(* Logix 5000 AddOnInstructionDefinition export Banner_K50Audible_PD_v4; software revision 33.00 *)

TYPE Banner_K50Audible_Advanced_PD_v4 :   // K50 Pro Audible Advanced
STRUCT
   PDI_Output_State : SINT;   // 0 = Inactive,1 = Active
   PDO_Animation : SINT;   // 0 = Off, 1 = Steady, 2 = Flash, 3 = 2 Color Flash, 4 = 50/50, 5 = 50/50 Rotate, 6 = Chase, 7 = Intensity Sweep, 8 = Color Sweep, 9 Sequence, 10 = Wave, 11 = Double Wave
   PDO_Direction : SINT;   // 0 = CCW, 1 = CW
   PDO_Pattern : SINT;   // 0 = Slow, 1 = Strobe, 2 = 3 Pulse, 3 = SOS, 4 = Random
   PDO_Speed : SINT;   // 0 = Slow, 1 = Medium, 2 = Fast, 3 = Custom
   PDO_Audio_Feedback : SINT;   // 0 = Off, 1 = On, 2 = Animation Pattern, 3 = Advanced Audible
   PDO_Off_Delay_Type : SINT;   // 0 = Leading Edge, 1 = Trailing Edge
   PDO_Off_Delay : DINT;   // 0 to 65535. Length of time before device returns to touch inactive after button press.
   PDO_Static_Sequence : SINT;   // 0 to 255. Value describing LED position
   PDO_Sequence_Start_Location : SINT;   // 0 = LED1, 1 = LED2, 2 = LED3, 3 = LED4, 4 = LED5, 5 = LED6, 6 = LED7, 7 = LED8
   PDO_Color_1 : SINT;   // 0 = Green, 1 = Red, 2 = Orange, 3 = Amber, 4 = Yellow, 5 = Lime Green, 6 = Spring Green, 7 = Cyan, 8 = Sky Blue, 9 = Blue, 10 = Violet, 11 = Magenta, 12 = Rose, 13 = White, 14 = Custom 1, 15 = Custom 2
   PDO_Color_1_Intensity : SINT;   // 0 = High, 1 = Medium, 2 = Low, 3 = Off, 4 = Custom
   PDO_Color_2 : SINT;   // 0 = Green, 1 = Red, 2 = Orange, 3 = Amber, 4 = Yellow, 5 = Lime Green, 6 = Spring Green, 7 = Cyan, 8 = Sky Blue, 9 = Blue, 10 = Violet, 11 = Magenta, 12 = Rose, 13 = White, 14 = Custom 1, 15 = Custom 2.
   PDO_Color_2_Intensity : SINT;   // 0 = High, 1 = Medium, 2 = Low, 3 = Off, 4 = Custom
   PDO_Audio_Volume : SINT;   // 1 = Low, 3 = High
   PDO_Audio_Type : SINT;   // 0 = Pulse, 1 = Wobble, 2 = Strobe, 3 = Whoop, 4 = Stacatto, 5 = Siren, 6 = Continuous 1, 7 = Continuous 2, 9 = Jingle, 10 = Melody 1, 11 = Melody 2, 12 = Melody 3, 13 Custom
END_STRUCT
END_TYPE

TYPE Banner_K50Audible_Four_PD_v4 :   // K50 Pro Audible Four State Full Logic
STRUCT
   PDI_Output_State : SINT;   // 0 = Inactive,1 = Active
   PDI_State : SINT;   // 0 = State 1, 1 = State 2, 2 = State 3, 3 = State 4
   PDO_Job_Input : SINT;   // 0 = State 1, 1 = State 2, 2 = State 3, 3 = State 4
END_STRUCT
END_TYPE

TYPE Banner_K50Audible_LED_v4 :   // LED Control Process Data for a K50 Pro Audible.
STRUCT
   Output_State : SINT;   // 0 = Inactive, 1 = Active.
   LED_1_Color : SINT;   // 0 = Green, 1 = Red, 2 = Orange, 3 = Amber, 4 = Yellow, 5 = Lime Green, 6 = Spring Green, 7 = Cyan, 8 = Sky Blue, 9 = Blue, 10 = Violet, 11 = Magenta, 12 = Rose, 13 = White, 14 = Custom 1, 15 = Custom 2.
   LED_1_Intensity : SINT;   // 0 to 10 (0 to 100%).
   LED_2_Color : SINT;   // 0 = Green, 1 = Red, 2 = Orange, 3 = Amber, 4 = Yellow, 5 = Lime Green, 6 = Spring Green, 7 = Cyan, 8 = Sky Blue, 9 = Blue, 10 = Violet, 11 = Magenta, 12 = Rose, 13 = White, 14 = Custom 1, 15 = Custom 2.
   LED_2_Intensity : SINT;   // 0 to 10 (0 to 100%).
   LED_3_Color : SINT;   // 0 = Green, 1 = Red, 2 = Orange, 3 = Amber, 4 = Yellow, 5 = Lime Green, 6 = Spring Green, 7 = Cyan, 8 = Sky Blue, 9 = Blue, 10 = Violet, 11 = Magenta, 12 = Rose, 13 = White, 14 = Custom 1, 15 = Custom 2.
   LED_3_Intensity : SINT;   // 0 to 10 (0 to 100%).
   LED_4_Color : SINT;   // 0 = Green, 1 = Red, 2 = Orange, 3 = Amber, 4 = Yellow, 5 = Lime Green, 6 = Spring Green, 7 = Cyan, 8 = Sky Blue, 9 = Blue, 10 = Violet, 11 = Magenta, 12 = Rose, 13 = White, 14 = Custom 1, 15 = Custom 2.
   LED_4_Intensity : SINT;   // 0 to 10 (0 to 100%).
   LED_5_Color : SINT;   // 0 = Green, 1 = Red, 2 = Orange, 3 = Amber, 4 = Yellow, 5 = Lime Green, 6 = Spring Green, 7 = Cyan, 8 = Sky Blue, 9 = Blue, 10 = Violet, 11 = Magenta, 12 = Rose, 13 = White, 14 = Custom 1, 15 = Custom 2.
   LED_5_Intensity : SINT;   // 0 to 10 (0 to 100%).
   LED_6_Color : SINT;   // 0 = Green, 1 = Red, 2 = Orange, 3 = Amber, 4 = Yellow, 5 = Lime Green, 6 = Spring Green, 7 = Cyan, 8 = Sky Blue, 9 = Blue, 10 = Violet, 11 = Magenta, 12 = Rose, 13 = White, 14 = Custom 1, 15 = Custom 2.
   LED_6_Intensity : SINT;   // 0 to 10 (0 to 100%).
   LED_7_Color : SINT;   // 0 = Green, 1 = Red, 2 = Orange, 3 = Amber, 4 = Yellow, 5 = Lime Green, 6 = Spring Green, 7 = Cyan, 8 = Sky Blue, 9 = Blue, 10 = Violet, 11 = Magenta, 12 = Rose, 13 = White, 14 = Custom 1, 15 = Custom 2.
   LED_7_Intensity : SINT;   // 0 to 10 (0 to 100%).
   LED_8_Color : SINT;   // 0 = Green, 1 = Red, 2 = Orange, 3 = Amber, 4 = Yellow, 5 = Lime Green, 6 = Spring Green, 7 = Cyan, 8 = Sky Blue, 9 = Blue, 10 = Violet, 11 = Magenta, 12 = Rose, 13 = White, 14 = Custom 1, 15 = Custom 2.
   LED_8_Intensity : SINT;   // 0 to 10 (0 to 100%).
   Audio_Feedback : SINT;   // 0 = Off, 1 = On, 2 = Pattern, 3 = Advanced Audible
   Audio_Volume : SINT;   // 1 = Low, 3 = High
   Audio_Type : SINT;   // 0 = Pulse, 1 = Wobble, 2 = Strobe, 3 = Whoop, 4 = Stacatto, 5 = Siren, 6 = Continuous 1, 7 = Continuous 2, 9 = Jingle, 10 = Melody 1, 11 = Melody 2, 12 = Melody 3, 13 Custom
END_STRUCT
END_TYPE

TYPE Banner_K50Audible_Multi_PD_v4 :   // K50 Pro Audible Multicolor Process Data
STRUCT
   PDI_Output_State : SINT;   // 0 = Inactive,1 = Active
   PDI_State : SINT;   // 0 = State 1, 1 = State 2, 2 = State 3, 3 = State 4
   PDO_State : SINT;   // 0 = State 1, 1 = State 2, 2 = State 3, 3 = State 4
END_STRUCT
END_TYPE

TYPE Banner_K50Audible_PDIO_v4 :   // UDT that records the converted prcoess data.
STRUCT
   PD_MultiColor_State : Banner_K50Audible_Multi_PD_v4;   // Only active when Operation Mode set to 0. State tells the light which of the four states it should be in. 0 = State 1, 1 = State 2, 2 = State 3, 3 = State 4.
   PD_FourState_Job_Input : Banner_K50Audible_Four_PD_v4;   // Only active when Operation Mode set to 1. Job Input tells the light how it should behave. 0 - Off, 1 = ON
   PD_Advanced : Banner_K50Audible_Advanced_PD_v4;   // Only active when Operation Mode set to 2.
   PD_LED : Banner_K50Audible_LED_v4;   // Only active when Operation Mode set to 3.
   PDO_DT : SINT[10];
   PDI_DT : SINT[2];
END_STRUCT
END_TYPE

ADD_ON_INSTRUCTION Banner_K50Audible_PD_v4   (* revision 4.0, vendor Banner Engineering *)
// Takes the raw SINT information and converts that data into actual information.
VAR_IN_OUT
   PDIO : Banner_K50Audible_PDIO_v4; {required}
END_VAR
VAR_INPUT
   Operation_Mode : SINT; {required}   // Linked from Parameters AOI or entered manually.
   Byte_Swap : BOOL; {required}
END_VAR
VAR
   PDO_Temp : SINT[10]; {access None}
   PDI_Temp : SINT[2]; {access None}
END_VAR

ROUTINE Logic   (* ladder *)
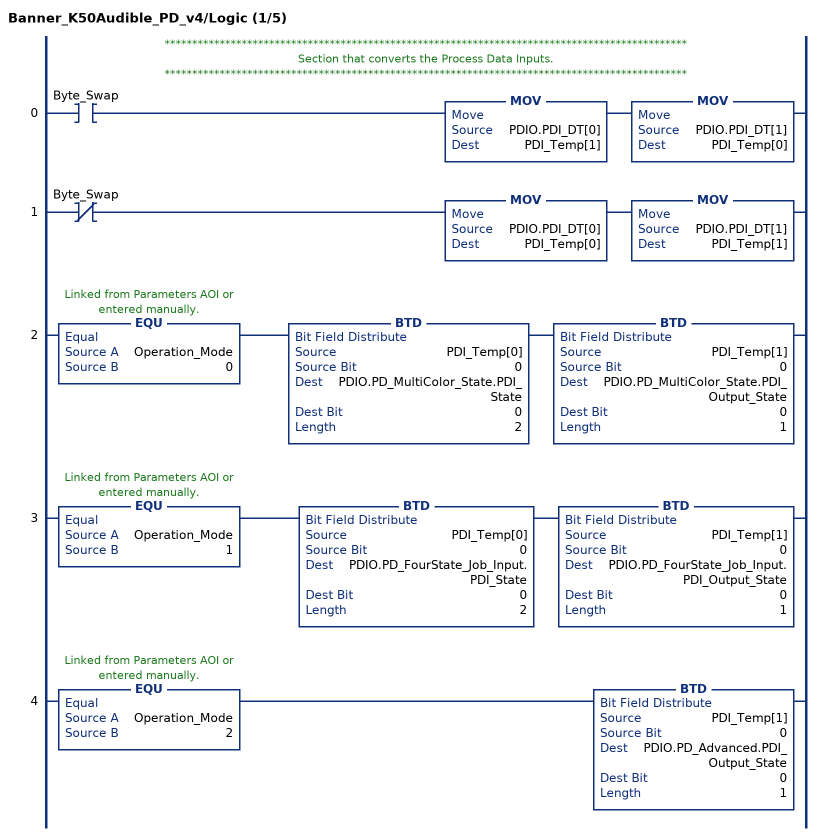
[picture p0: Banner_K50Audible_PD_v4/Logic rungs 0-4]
   // ***********************************************************************************************
   // Section that converts the Process Data Inputs.
   // ***********************************************************************************************
   0: XIC(Byte_Swap)MOV(PDIO.PDI_DT[0],PDI_Temp[1])MOV(PDIO.PDI_DT[1],PDI_Temp[0]);
   1: XIO(Byte_Swap)MOV(PDIO.PDI_DT[0],PDI_Temp[0])MOV(PDIO.PDI_DT[1],PDI_Temp[1]);
   2: EQU(Operation_Mode,0)BTD(PDI_Temp[0],0,PDIO.PD_MultiColor_State.PDI_State,0,2)BTD(PDI_Temp[1],0,PDIO.PD_MultiColor_State.PDI_Output_State,0,1);
   3: EQU(Operation_Mode,1)BTD(PDI_Temp[0],0,PDIO.PD_FourState_Job_Input.PDI_State,0,2)BTD(PDI_Temp[1],0,PDIO.PD_FourState_Job_Input.PDI_Output_State,0,1);
   4: EQU(Operation_Mode,2)BTD(PDI_Temp[1],0,PDIO.PD_Advanced.PDI_Output_State,0,1);
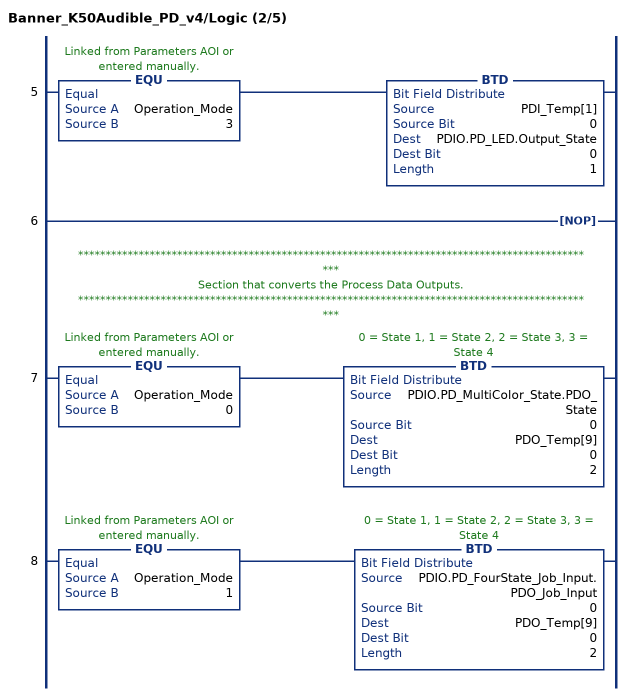
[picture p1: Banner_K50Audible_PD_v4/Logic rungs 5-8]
   5: EQU(Operation_Mode,3)BTD(PDI_Temp[1],0,PDIO.PD_LED.Output_State,0,1);
   6: NOP();
   // ***********************************************************************************************
   // Section that converts the Process Data Outputs.
   // ***********************************************************************************************
   7: EQU(Operation_Mode,0)BTD(PDIO.PD_MultiColor_State.PDO_State,0,PDO_Temp[9],0,2);
   8: EQU(Operation_Mode,1)BTD(PDIO.PD_FourState_Job_Input.PDO_Job_Input,0,PDO_Temp[9],0,2);
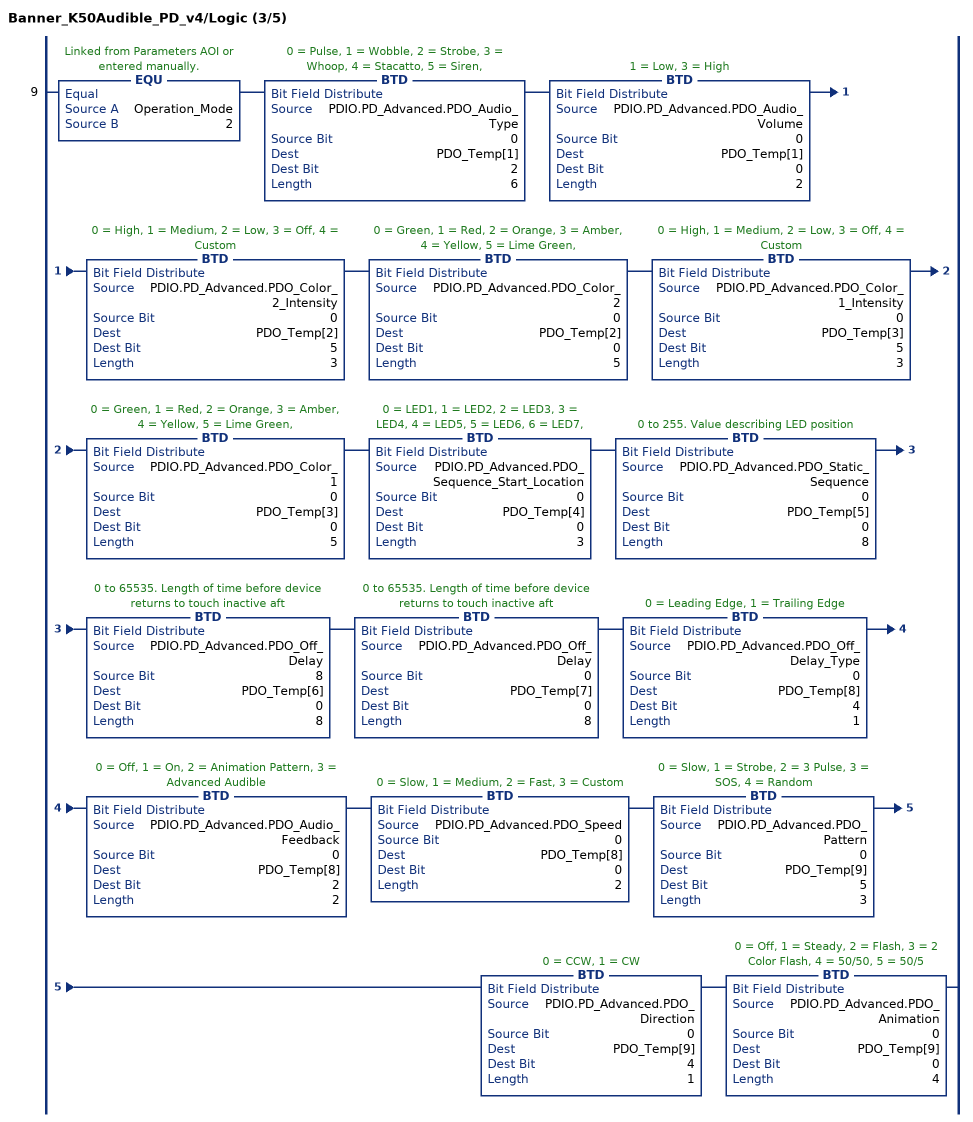
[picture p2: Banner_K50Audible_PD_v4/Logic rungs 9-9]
   9: EQU(Operation_Mode,2)BTD(PDIO.PD_Advanced.PDO_Audio_Type,0,PDO_Temp[1],2,6)BTD(PDIO.PD_Advanced.PDO_Audio_Volume,0,PDO_Temp[1],0,2)BTD(PDIO.PD_Advanced.PDO_Color_2_Intensity,0,PDO_Temp[2],5,3)BTD(PDIO.PD_Advanced.PDO_Color_2,0,PDO_Temp[2],0,5)BTD(PDIO.PD_Advanced.PDO_Color_1_Intensity,0,PDO_Temp[3],5,3)BTD(PDIO.PD_Advanced.PDO_Color_1,0,PDO_Temp[3],0,5)BTD(PDIO.PD_Advanced.PDO_Sequence_Start_Location,0,PDO_Temp[4],0,3)BTD(PDIO.PD_Advanced.PDO_Static_Sequence,0,PDO_Temp[5],0,8)BTD(PDIO.PD_Advanced.PDO_Off_Delay,8,PDO_Temp[6],0,8)BTD(PDIO.PD_Advanced.PDO_Off_Delay,0,PDO_Temp[7],0,8)BTD(PDIO.PD_Advanced.PDO_Off_Delay_Type,0,PDO_Temp[8],4,1)BTD(PDIO.PD_Advanced.PDO_Audio_Feedback,0,PDO_Temp[8],2,2)BTD(PDIO.PD_Advanced.PDO_Speed,0,PDO_Temp[8],0,2)BTD(PDIO.PD_Advanced.PDO_Pattern,0,PDO_Temp[9],5,3)BTD(PDIO.PD_Advanced.PDO_Direction,0,PDO_Temp[9],4,1)BTD(PDIO.PD_Advanced.PDO_Animation,0,PDO_Temp[9],0,4);
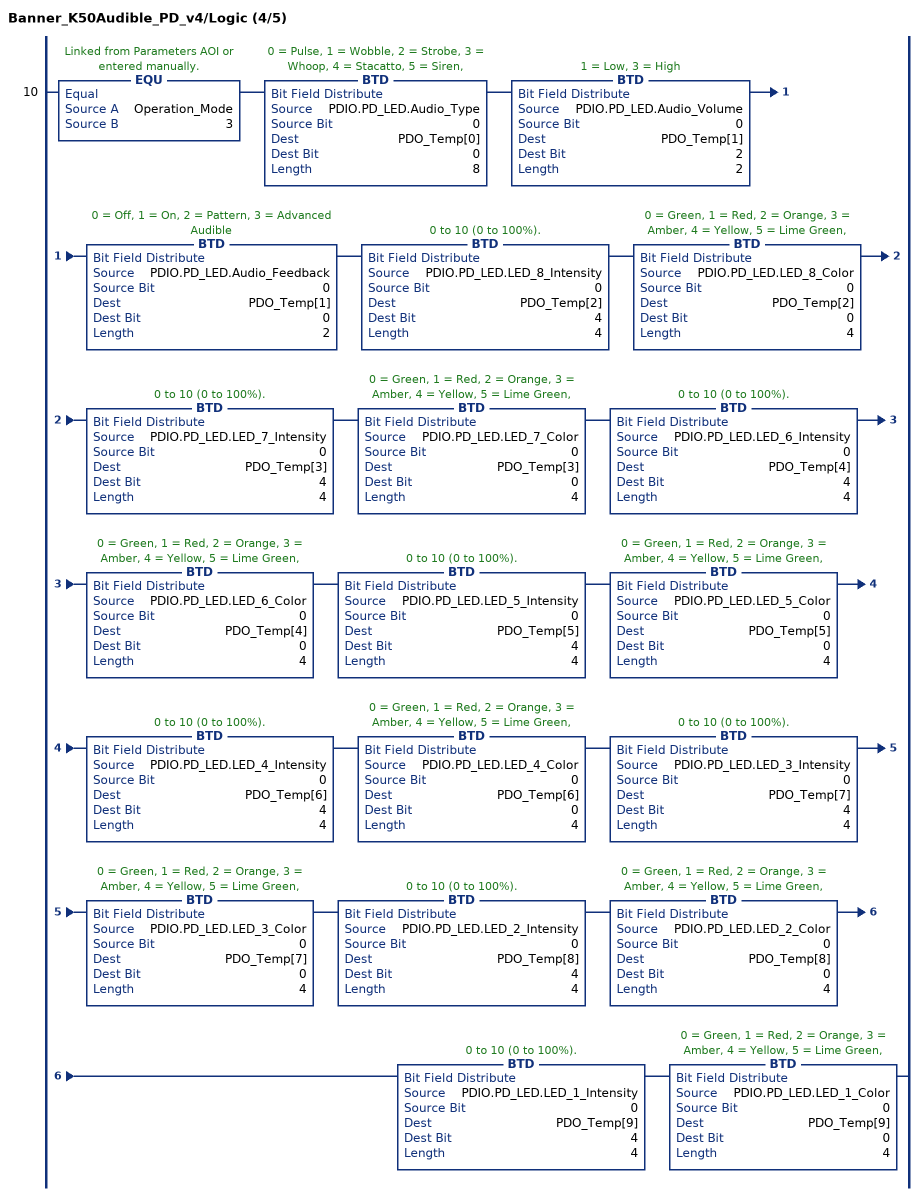
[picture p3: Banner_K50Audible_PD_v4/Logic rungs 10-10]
   10: EQU(Operation_Mode,3)BTD(PDIO.PD_LED.Audio_Type,0,PDO_Temp[0],0,8)BTD(PDIO.PD_LED.Audio_Volume,0,PDO_Temp[1],2,2)BTD(PDIO.PD_LED.Audio_Feedback,0,PDO_Temp[1],0,2)BTD(PDIO.PD_LED.LED_8_Intensity,0,PDO_Temp[2],4,4)BTD(PDIO.PD_LED.LED_8_Color,0,PDO_Temp[2],0,4)BTD(PDIO.PD_LED.LED_7_Intensity,0,PDO_Temp[3],4,4)BTD(PDIO.PD_LED.LED_7_Color,0,PDO_Temp[3],0,4)BTD(PDIO.PD_LED.LED_6_Intensity,0,PDO_Temp[4],4,4)BTD(PDIO.PD_LED.LED_6_Color,0,PDO_Temp[4],0,4)BTD(PDIO.PD_LED.LED_5_Intensity,0,PDO_Temp[5],4,4)BTD(PDIO.PD_LED.LED_5_Color,0,PDO_Temp[5],0,4)BTD(PDIO.PD_LED.LED_4_Intensity,0,PDO_Temp[6],4,4)BTD(PDIO.PD_LED.LED_4_Color,0,PDO_Temp[6],0,4)BTD(PDIO.PD_LED.LED_3_Intensity,0,PDO_Temp[7],4,4)BTD(PDIO.PD_LED.LED_3_Color,0,PDO_Temp[7],0,4)BTD(PDIO.PD_LED.LED_2_Intensity,0,PDO_Temp[8],4,4)BTD(PDIO.PD_LED.LED_2_Color,0,PDO_Temp[8],0,4)BTD(PDIO.PD_LED.LED_1_Intensity,0,PDO_Temp[9],4,4)BTD(PDIO.PD_LED.LED_1_Color,0,PDO_Temp[9],0,4);
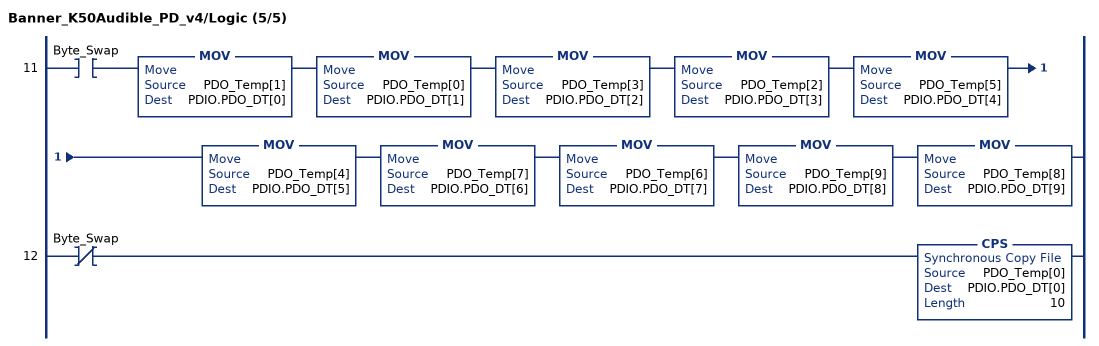
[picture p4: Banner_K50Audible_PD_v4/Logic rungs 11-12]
   11: XIC(Byte_Swap)MOV(PDO_Temp[1],PDIO.PDO_DT[0])MOV(PDO_Temp[0],PDIO.PDO_DT[1])MOV(PDO_Temp[3],PDIO.PDO_DT[2])MOV(PDO_Temp[2],PDIO.PDO_DT[3])MOV(PDO_Temp[5],PDIO.PDO_DT[4])MOV(PDO_Temp[4],PDIO.PDO_DT[5])MOV(PDO_Temp[7],PDIO.PDO_DT[6])MOV(PDO_Temp[6],PDIO.PDO_DT[7])MOV(PDO_Temp[9],PDIO.PDO_DT[8])MOV(PDO_Temp[8],PDIO.PDO_DT[9]);
   12: XIO(Byte_Swap)CPS(PDO_Temp[0],PDIO.PDO_DT[0],10);
END_ROUTINE
END_ADD_ON_INSTRUCTION
